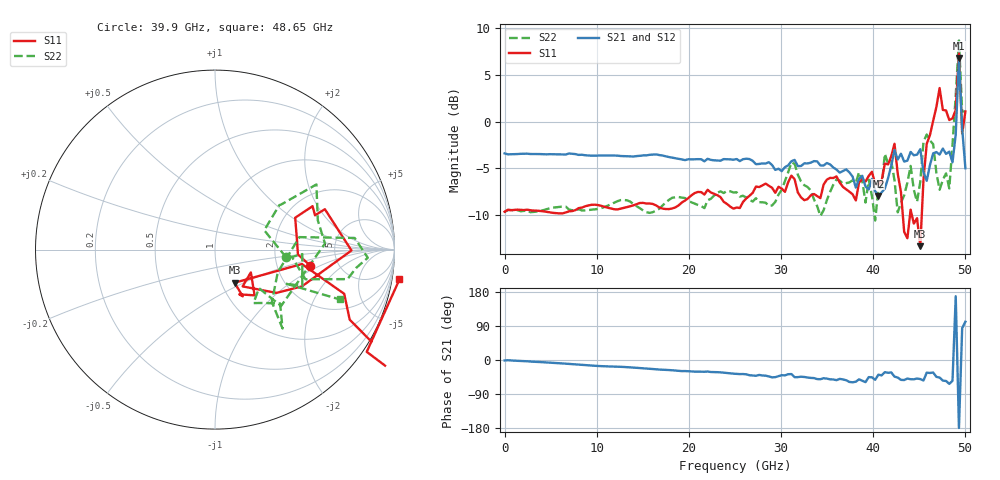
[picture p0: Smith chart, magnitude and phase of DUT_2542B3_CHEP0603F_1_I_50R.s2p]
! 10/31/2025 3:28:55 PM
! C:\MESURES\046-TRL-DUT-CHEP0603\DUT\DUT-2542B3-CHEP0603F-1-I.S2P
! CHANNEL.1 Sparams
! TR.MEASUREMENT
! CORRECTED.DATA
! RF.CORRECTION: CAL.A: FULL.TWO.PORT.CALCAL.A: Port 1,4
! AVERAGING.OFF
! IF.BANDWIDTH: 500HZ
! SWEEPTYPE:  FREQ.SWEEP(Linear)
! Reference Plane Port Info
! PORT:  PORT1  PORT4
! DISTANCE:  0  m  0  m
! TIME:  0  s  0  s
! PHASE.OFFSET:  0  deg.  0  deg.
! LOSS:  0  dB  0  dB
! REF.LOSS:  0  dB  0  dB
! REF.FREQ:  0  Hz  0  Hz
! Power Info
! POWER:  -10  dBm  -10  dBm
! EFF.POWER:  -10  dBm  -10  dBm
! SOURCE.ATTEN:  0  dB  0  dB
! TEST.ATTEN:  0  dB  0  dB
! PORTZ: Port1:50 Port4:50
# GHZ S RI R 50
! FREQ.GHZ  S11RE  S11IM  S41RE  S41IM  S14RE  S14IM  S44RE  S44IM
!; PortSelection: Port_14 (1-->1,4-->4)
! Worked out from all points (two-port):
!   144 points, 10 MHz to 50.05 GHz, reference 50 ohm
!   highest |S21| = 6.83 dB at 49.35 GHz (marker M1); lowest = -8.0 dB at 40.6 GHz (marker M2)
!   |S21| within 3 dB of the highest: 49.23 GHz to 49.49 GHz (266.1 MHz wide, 0.539 % of centre)
!   lowest |S11| = -13.4 dB at 45.15 GHz (marker M3), VSWR 1.55, Z = 57.6 - j22.3 ohm
!   |S11| at or under -10 dB: 43.25 GHz to 44.04 GHz (786.5 MHz wide, 1.8 % of centre); 44.23 GHz to 45.32 GHz (1.085 GHz wide, 2.42 % of centre)
!   |S22| runs from -10.6 to 8.7 dB; largest |S21 - S12| = 0.029
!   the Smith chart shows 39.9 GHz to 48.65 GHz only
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0.01  0.328 0.0153  0.6751 -0.0149  0.6757 -0.0152  0.3276 0.015
8.4088  0.3416 -0.0525  0.6474 -0.1484  0.6461 -0.1464  0.3295 -0.0519
16.8076  0.3405 -0.0617  0.5981 -0.2825  0.5978 -0.2793  0.3289 -0.0884
25.2064  0.3389 -0.0684  0.5045 -0.3767  0.5061 -0.3739  0.4087 -0.0859
33.6052  0.3863 -0.134  0.4129 -0.4541  0.4165 -0.4517  0.3765 -0.0696
37.8046  0.3879 -0.1239  0.2626 -0.4333  0.2652 -0.4315  0.4409 -0.2009
40.6042  0.4574 0.0441  0.3106 -0.2493  0.3118 -0.247  0.3587 0.2482
41.3041  0.5435 0.2418  0.3701 -0.2321  0.371 -0.2297  0.565 0.3631
42.004  0.6123 0.2251  0.4866 -0.3145  0.4894 -0.3095  0.6127 0.0341
42.35395  0.7604 -0.00489  0.5084 -0.4877  0.5121 -0.4828  0.3683 -0.3142
42.7039  0.4845 -0.2048  0.4325 -0.4524  0.4341 -0.4504  0.245 -0.2149
44.1037  0.2205 -0.2549  0.4353 -0.5321  0.4397 -0.5258  0.3763 -0.4396
45.15355  0.1089 -0.1849  0.4541 -0.5469  0.458 -0.5396  0.4708 0.0695
45.85345  0.7198 -0.2463  0.4021 -0.2642  0.4048 -0.259  0.8513 -0.0454
47.25325  1.054 -1.087  0.4599 -0.4809  0.4654 -0.4734  0.4286 -0.0409
47.6032  0.5306 -1.026  0.4163 -0.5833  0.4214 -0.5769  0.4867 -0.025
47.95315  0.9475 -0.6465  0.3814 -0.5525  0.3875 -0.5478  0.4866 -0.2033
48.65305  1.028 -0.1662  0.348 -0.495  0.3527 -0.4915  0.6945 -0.2774
49.003  1.122 -0.2744  -0.8324 0.1734  -0.8326 0.1624  1.302 0.464
49.35295  2.306 -0.2504  -2.196 -0.0242  -2.183 -0.0508  2.466 1.163
49.7029  0.8444 -0.1776  0.0944 0.9141  0.0807 0.9131  1.094 -0.3048
50.05285  1.077 -0.3509  -0.107 0.5518  -0.1134 0.5529  1.118 -0.1664
